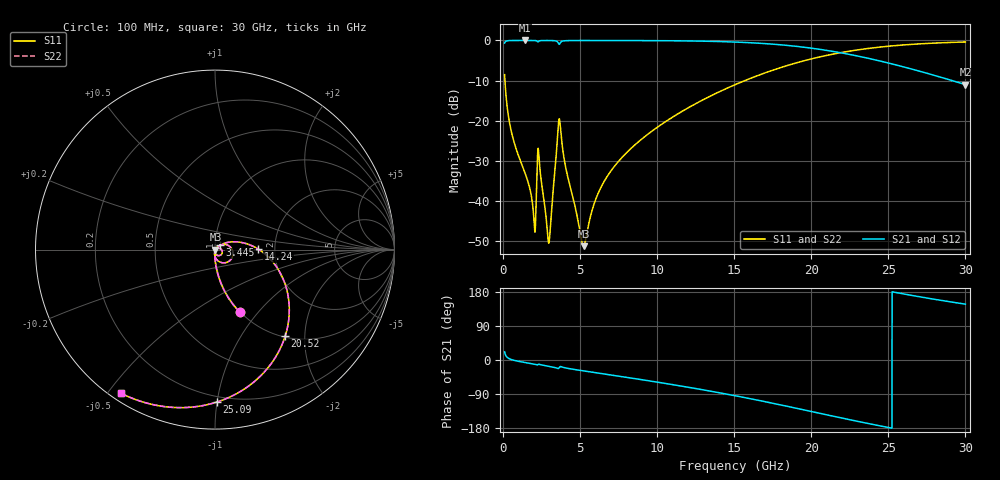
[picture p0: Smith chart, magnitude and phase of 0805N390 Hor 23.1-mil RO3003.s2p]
# GHz S MA R 50
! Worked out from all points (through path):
!   3201 points, 100 MHz to 30 GHz, reference 50 ohm
!   highest |S21| = -0.01 dB at 1.408 GHz (marker M1); lowest = -11.0 dB at 30 GHz (marker M2)
!   group delay of S21, straight-line fit = 20.7 ps
!   lowest |S11| = -51.2 dB at 5.22 GHz (marker M3), VSWR 1.01, Z = 50.2 - j0.122 ohm
!   |S11| at or under -10 dB: 121.2 MHz to 15.69 GHz (15.57 GHz wide, 197 % of centre)
!   |S22| runs from -51.2 to -0.4 dB; largest |S21 - S12| = 0
!   S11 on the Smith chart (normalised r, x): 100 MHz: 0.99, -0.81; 3.445 GHz: 1.05, +0.05; 14.24 GHz: 1.63, +0.01; 20.52 GHz: 1.02, -1.60; 25.09 GHz: 0.16, -1.00; 30 GHz: 0.03, -0.54
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0.1  0.3745 -68.5  0.9269 21.4  0.9269 21.4  0.3745 -68.5
0.5485  0.07171 -88.5  0.9968 1.1  0.9968 1.1  0.07171 -88.5
1.408125  0.02282 -93.9  0.9987 -6.5  0.9987 -6.5  0.02282 -93.9
2.006125  0.005801 -74.3  0.9973 -10.9  0.9973 -10.9  0.005801 -74.3
2.351844  0.03101 -73.7  0.9851 -11.5  0.9851 -11.5  0.03101 -73.7
2.959188  0.003 -26.3  0.9969 -16.4  0.9969 -16.4  0.003 -26.3
3.09  0.005527 32.4  0.9963 -17.4  0.9963 -17.4  0.005527 32.4
3.445063  0.03664 41.7  0.9825 -20.9  0.9825 -20.9  0.03664 41.7
3.585219  0.08665 9.8  0.9256 -22.5  0.9256 -22.5  0.08665 9.8
3.706688  0.08942 -56.0  0.9285 -17.3  0.9285 -17.3  0.08942 -56.0
5.089563  0.003248 -58.1  0.997 -27.9  0.997 -27.9  0.003248 -58.1
5.220375  0.002749 -26.2  0.9971 -28.7  0.9971 -28.7  0.002749 -26.2
5.958531  0.009873 41.3  0.9971 -33.2  0.9971 -33.2  0.009873 41.3
6.75275  0.02024 44.4  0.9969 -38.0  0.9969 -38.0  0.02024 44.4
10.06978  0.08462 28.9  0.9927 -58.8  0.9927 -58.8  0.08462 28.9
14.23709  0.2394 0.9  0.9658 -88.0  0.9658 -88.0  0.2394 0.9
15.05  0.281 -5.2  0.9543 -94.2  0.9543 -94.2  0.281 -5.2
20.03956  0.591 -46.8  0.7992 -136.2  0.7992 -136.2  0.591 -46.8
20.51609  0.6212 -51.0  0.776 -140.4  0.776 -140.4  0.6212 -51.0
25.01978  0.8472 -88.8  0.5222 -178.3  0.5222 -178.3  0.8472 -88.8
25.08519  0.8495 -89.3  0.5185 -178.8  0.5185 -178.8  0.8495 -89.3
30  0.9561 -123.1  0.2818 147.4  0.2818 147.4  0.9561 -123.1
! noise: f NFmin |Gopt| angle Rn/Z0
0.1  0.0004641  0.8698  0.783  0.0007672
3.417  0.0162  0.8732  18.91  0.02682
6.743  0.01017  0.6549  36.73  0.005081
10.06  0.01376  0.6349  53.41  0.005734
13.39  0.01798  0.6393  68.94  0.00654
16.7  0.02305  0.6572  83.3  0.007405
20.03  0.02952  0.6855  96.78  0.008388
23.35  0.03819  0.7227  109.6  0.009549
26.67  0.05057  0.7674  122.2  0.01092
30  0.06936  0.8167  134.8  0.01237
